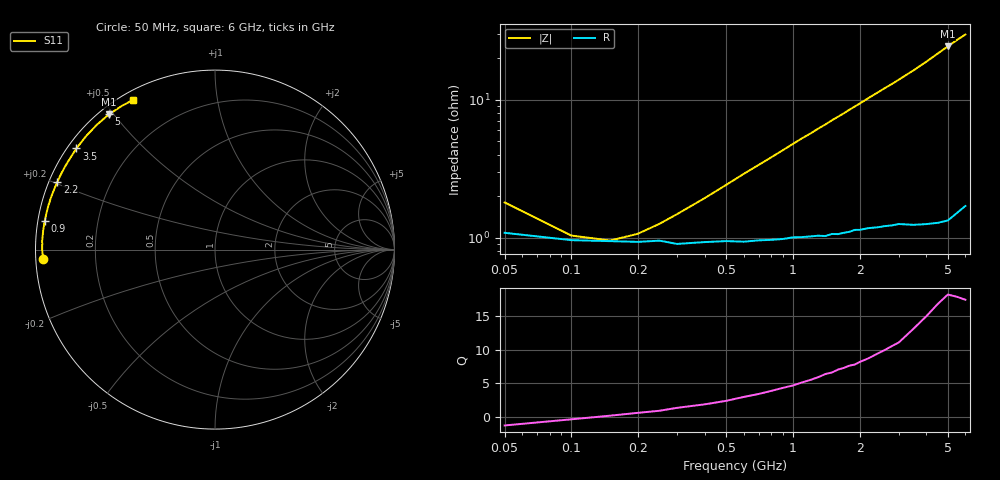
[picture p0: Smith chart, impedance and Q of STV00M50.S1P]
! SIEMENS Discrete & RF Semiconductors
! BA892
! Si PIN Diode in SCD-80
! IF = 0.5 mA
! S-Parameters:  September  1997
# GHz  S  MA  R  50
!  f  S11
! GHz  MAG  ANG
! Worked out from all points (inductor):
!   34 points, 50 MHz to 6 GHz, reference 50 ohm
!   read as one part to ground: L = 743 pH near 700 MHz
!   highest Q = 17.9 at 5 GHz (marker M1), where L = 774 pH
!   S11 on the Smith chart (normalised r, x): 50 MHz: 0.02, -0.03; 900 MHz: 0.02, +0.08; 2.2 GHz: 0.02, +0.21; 3.5 GHz: 0.02, +0.33; 5 GHz: 0.03, +0.49; 6 GHz: 0.03, +0.59
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0.05  0.9575 -176.7
0.1  0.9623 -179.1
0.15  0.9629 179.7
0.2  0.9633 178.8
0.25  0.9626 178.1
0.3  0.9645 177.3
0.6  0.9633 173.7
0.8  0.9623 171.5
0.9  0.9618 170.4
1.1  0.9607 168.2
1.2  0.9604 167.2
1.3  0.96 166.1
1.4  0.9603 165.1
1.5  0.959 164.0
1.6  0.9592 163.0
1.7  0.9584 162.0
1.8  0.9579 160.9
2  0.9568 158.9
2.2  0.9558 156.8
2.4  0.9556 154.8
2.6  0.9551 152.8
2.8  0.9549 150.9
3.5  0.9561 143.9
4  0.9569 138.7
4.5  0.9576 133.3
5  0.9577 128.1
5.5  0.9542 123.1
6  0.9509 118.6
